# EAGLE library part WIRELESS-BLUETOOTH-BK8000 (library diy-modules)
Bluetooth Audio Module based on BK8000L chip More details available here: http://www.electrodragon.com/w/BK8000L Click here to find device on ebay.com
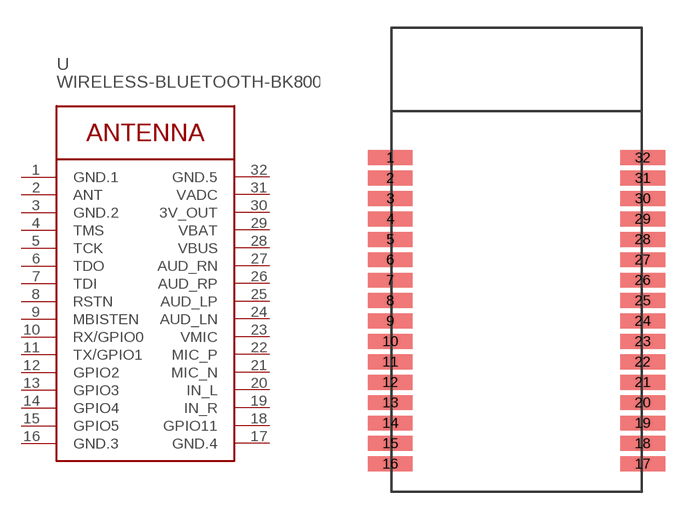
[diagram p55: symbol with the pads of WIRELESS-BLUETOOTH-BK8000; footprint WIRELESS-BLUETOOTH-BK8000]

Designator prefix -

## WIRELESS-BLUETOOTH-BK8000  [WIRELESS-BLUETOOTH-BK8000]
1  GND.1  pwr
2  ANT  pas
3  GND.2  pwr
4  TMS
5  TCK
6  TDO
7  TDI
8  RSTN
9  MBISTEN
10  RX/GPIO0
11  TX/GPIO1
12  GPIO2
13  GPIO3
14  GPIO4
15  GPIO5
16  GND.3  pwr
17  GND.4  pwr
18  GPIO11
19  IN_R  in
20  IN_L  in
21  MIC_N  in
22  MIC_P  in
23  VMIC  pas
24  AUD_LN  out
25  AUD_LP  out
26  AUD_RP  out
27  AUD_RN  out
28  VBUS  pas
29  VBAT  pas
30  3V_OUT  pwr
31  VADC  pwr
32  GND.5  pwr

## Footprint WIRELESS-BLUETOOTH-BK8000 (pad centres in mm)
Bluetooth Audio Module based on BK8000L chip
smd 2.4 x 0.8: 1 -6.8,5.5; 2 -6.8,4.4; 3 -6.8,3.3; 4 -6.8,2.2; 5 -6.8,1.1; 6 -6.8,0; 7 -6.8,-1.1; 8 -6.8,-2.2; 9 -6.8,-3.3; 10 -6.8,-4.4; 11 -6.8,-5.5; 12 -6.8,-6.6; 13 -6.8,-7.7; 14 -6.8,-8.8; 15 -6.8,-9.9; 16 -6.8,-11; 17 6.8,-11; 18 6.8,-9.9; 19 6.8,-8.8; 20 6.8,-7.7; 21 6.8,-6.6; 22 6.8,-5.5; 23 6.8,-4.4; 24 6.8,-3.3; 25 6.8,-2.2; 26 6.8,-1.1; 27 6.8,0; 28 6.8,1.1; 29 6.8,2.2; 30 6.8,3.3; 31 6.8,4.4; 32 6.8,5.5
